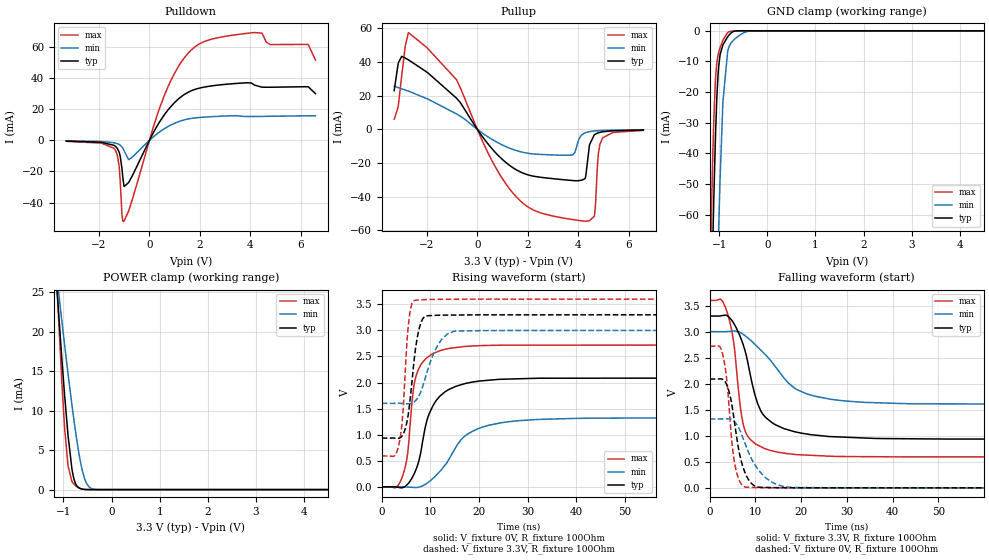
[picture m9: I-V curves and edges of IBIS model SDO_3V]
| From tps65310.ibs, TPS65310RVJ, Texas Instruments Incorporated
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[Model]   SDO_3V
Model_type   Output
Polarity   Non-Inverting
Vmeas = 1.65
Vref = 1.65
Cref = 15pF
Rref = 50
|   typ   min   max
|   (slow PVT)   (Fast PVT)   (nom PVT)
C_comp   2.409p   2.166p   2.464p
|C_comp (Hi state)   2.409p   2.166p   2.464p
|C_comp (Low state)   2.989p   2.727p   3.127p
[Voltage Range]   3.3   3   3.6
[Temperature Range]   27   175   -40
[Pullup Reference]   3.3   3   3.6
[Pulldown Reference]   -0   -0   -0
[Power Clamp Reference]   3.3   3   3.6
[GND Clamp Reference]   -0   -0   -0
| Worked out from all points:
|   slope of the pulldown table from 0 to 0.495 V, typ, clamps not added: 35.1 ohm
|   slope of the pullup table from 0 to 0.495 V, typ, clamps not added: 49.6 ohm
|   GND clamp passes 1 mA (typ) near -0.77 V on its own axis
|   POWER clamp passes 1 mA (typ) near -0.76 V on its own axis
|   falling waveform, V_fixture 3.3V, R_fixture 100Ohm: 20-80 % time 4.68ns typ, 8.9ns min, 2.55ns max; typ from 3.3 V to 0.936 V
|   rising waveform, V_fixture 0V, R_fixture 100Ohm: 20-80 % time 3.96ns typ, 6.87ns min, 2.06ns max; typ from 0 V to 2.09 V
|   rising waveform, V_fixture 3.3V, R_fixture 100Ohm: 20-80 % time 1.75ns typ, 3.29ns min, 1.22ns max; typ from 0.936 V to 3.3 V
|   falling waveform, V_fixture 0V, R_fixture 100Ohm: 20-80 % time 2.53ns typ, 4.58ns min, 1.73ns max; typ from 2.09 V to 0 V
[Pulldown]
|   Voltage   I(typ)   I(min)   I(max)
-3.3V     -468.4uA   -301.4uA   -623.8uA
-1.379V   -3.489mA   -1.642mA   -5.683mA
-1.211V   -7.228mA   -2.597mA   -15.53mA
-1.082V   -19.42mA   -4.376mA   -48.8mA
-1.013V   -29.05mA   -6.35mA    -52.05mA
-825mV    -27.1mA    -12.47mA   -45.43mA
561mV     15.7mA     7.157mA    27.55mA
1.739V    32.37mA    14.28mA    59.22mA
4.462V    34.2mA     15.4mA     68.97mA
4.798V    34.15mA    15.48mA    61.56mA
6.303V    34.44mA    15.79mA    61.62mA
6.59V     30mA       15.84mA    51.67mA
[GND Clamp]
|   Voltage   I(typ)   I(min)   I(max)
-3.3V     -2.142A    -2.212A    -2.12A
-1.231V   -144.3mA   -231.1mA   -112.3mA
-1.152V   -81.24mA   -165.3mA   -51.47mA
-1.132V   -67.01mA   -149.5mA   -38.93mA
-1.082V   -36.29mA   -111.8mA   -16.77mA
-1.053V   -22.7mA    -90.73mA   -10.66mA
-1.013V   -11.7mA    -65.08mA   -7.082mA
-924mV    -4.546mA   -23.13mA   -3.062mA
-825mV    -1.949mA   -6.652mA   -553.1uA
-795.3mV  -1.357mA   -5.177mA   -296.8uA
-339.9mV  0A         -50.26uA   0A
6.59V     0A         0A         0A
[Pullup]
|   Voltage   I(typ)   I(min)   I(max)
-3.3V     22.98mA    25.57mA    5.991mA
-3.132V   39.63mA    24.76mA    14.78mA
-2.736V   41.3mA     22.7mA     57.51mA
-825mV    18.5mA     9.135mA    29.47mA
1.531V    -23.91mA   -12.53mA   -39.86mA
3.779V    -30.41mA   -15.2mA    -53.61mA
4.303V    -27.82mA   -1.911mA   -54.65mA
4.452V    -9.19mA    -1.348mA   -54.28mA
4.65V     -3.212mA   -958.9uA   -51.06mA
4.798V    -2.085mA   -785.7uA   -15.32mA
4.966V    -1.479mA   -651.1uA   -5.208mA
6.59V     -379uA     -242.2uA   -623.2uA
[POWER Clamp]
|   Voltage   I(typ)   I(min)   I(max)
-3.3V     263.4mA    157mA      405.9mA
-1.201V   31.11mA    30.46mA    33.72mA
-1.033V   16.51mA    21.31mA    13.55mA
-973.5mV  11.78mA    18.19mA    7.65mA
-904.2mV  6.841mA    14.65mA    2.985mA
-825mV    2.674mA    10.79mA    1.052mA
-795.3mV  1.702mA    9.416mA    793.3uA
-735.9mV  613uA      6.824mA    458uA
-656.7mV  152.3uA    3.853mA    168.1uA
-518.1mV  8.889uA    791.9uA    6.343uA
-330mV    25.34nA    21.38uA    0A
6.59V     0A         0A         0A
[Ramp]
R_load = 100
|   typ   min   max
dV/dt_r   1.25313/3.94931e-09   0.793386/6.83878e-09   1.63259/2.05924e-09
dV/dt_f   1.41861/4.67857e-09   0.838706/8.81846e-09   1.80411/2.55497e-09
[Falling Waveform]
V_fixture = 3.3V
V_fixture_min = 3V
V_fixture_max = 3.6V
R_fixture = 100Ohm
C_fixture = 0F
|   Time   V(typ)   V(min)   V(max)
0s        3.3V       3V         3.6V
2.917ns   3.31V      2.999V     3.569V
5.42ns    3.137V     3.013V     2.679V
6.691ns   2.902V     2.981V     1.567V
7.558ns   2.686V     2.935V     1.149V
9.938ns   1.775V     2.753V     851.9mV
12.07ns   1.37V      2.567V     753.1mV
19.06ns   1.069V     1.888V     637.8mV
28.15ns   978.3mV    1.682V     603.3mV
100ns     935.6mV    1.602V     593.1mV
[Rising Waveform]
V_fixture = 0V
V_fixture_min = 0V
V_fixture_max = 0V
R_fixture = 100Ohm
C_fixture = 0F
|   Time   V(typ)   V(min)   V(max)
0s        1.001nV    588.4nV    661.7pV
3.892ns   -16.94mV   384.9uV    116.5mV
5.213ns   42.44mV    -3.005mV   568.1mV
5.791ns   105.5mV    -6.287mV   1.149V
7.359ns   415.8mV    -9.501mV   2.211V
9.418ns   1.319V     77.79mV    2.485V
12.07ns   1.749V     310.3mV    2.614V
17.43ns   1.988V     998.5mV    2.695V
26.34ns   2.068V     1.252V     2.718V
100ns     2.089V     1.322V     2.721V
[Rising Waveform]
V_fixture = 3.3V
V_fixture_min = 3V
V_fixture_max = 3.6V
R_fixture = 100Ohm
C_fixture = 0F
|   Time   V(typ)   V(min)   V(max)
0s        935.6mV    1.602V     593.1mV
3.652ns   935mV      1.604V     870.4mV
4.427ns   1.016V     1.599V     1.513V
5.377ns   1.347V     1.595V     3.012V
6.609ns   2.39V      1.627V     3.572V
7.645ns   3.021V     1.747V     3.586V
8.757ns   3.262V     2.028V     3.59V
11.56ns   3.291V     2.724V     3.596V
14.74ns   3.295V     2.981V     3.598V
100ns     3.3V       3V         3.6V
[Falling Waveform]
|Gnd
V_fixture = 0V
V_fixture_min = 0V
V_fixture_max = 0V
R_fixture = 100Ohm
C_fixture = 0F
|   Time   V(typ)   V(min)   V(max)
0s        2.089V     1.322V     2.721V
2.841ns   2.085V     1.325V     2.566V
3.652ns   1.995V     1.325V     2.148V
4.886ns   1.579V     1.306V     854.5mV
5.377ns   1.295V     1.275V     520.4mV
6.532ns   652.9mV    1.119V     131.1mV
7.797ns   279.8mV    838.9mV    13.78mV
11.56ns   9.973mV    251mV      3.499mV
16.89ns   2.63mV     15.11mV    1.515mV
100ns     13.37nV    745.8nV    4.598nV
